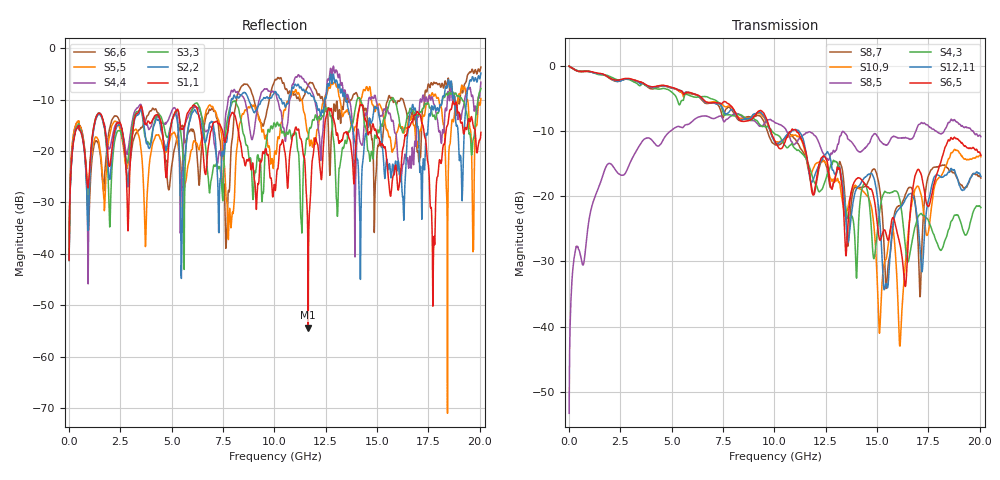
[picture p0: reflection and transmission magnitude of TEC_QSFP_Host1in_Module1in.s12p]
!!  This file represents Tyco Electronics parts only.  Due to internal design and materials, it should not  !!
!!  be used for products manufactured by companies other than Tyco Electronics.  !!
!! FILE NAME: TEC_QSFP_Host1in_Module1in.s12p
!! PART DESCRIPTION: Tyco Electronics QSFP P/N 1761987-9
!! PCB DESCRIPTION: Host Board FR4 with 1.5 inch microstrip, Module Board FR4 with 1.5 inch microstrip
!! FILE DESCRIPTION: 12 Port, S-Parameter, Measured Channel
!! FILE REVISION: Revision 2, 3/12/2008
!! FILE FREQUENCY RANGE: DC to 20.05 GHz in 12.50 MHz frequency steps
!! PORT DEFINITIONS:
!! Port  1  ----->  Host	Pin 14, RX3+	Module  <-----  Port  2
!! Port  3  ----->  Host	Pin 15, RX3-	Module  <-----  Port  4
!! Port  5  ----->  Host	Pin 21, RX2-	Module  <-----  Port  6
!! Port  7  ----->  Host	Pin 22, RX2+	Module  <-----  Port  8
!! Port  9  ----->  Host	Pin 24, RX4-	Module  <-----  Port  10
!! Port  11  ----->  Host	Pin 25, RX4+	Module  <-----  Port  12
# HZ S MA R 50.00
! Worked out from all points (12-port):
!   1604 points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, 12.5 MHz to 20.05 GHz, reference 50 ohm
!   strongest paths, dB at 12.5 MHz, 5.025 GHz, 10.04 GHz, 15.05 GHz, 20.05 GHz:
!     S6,5: 0.0, -3.3, -11.7, -25.4, -13.7
!     S12,11: -0.1, -3.4, -11.8, -21.1, -17.0
!     S4,3: -0.1, -4.1, -10.5, -24.2, -21.8
!     S8,5: -53.3, -9.8, -8.7, -11.0, -10.9
!     S10,9: -0.1, -3.4, -11.6, -36.5, -13.9
!     S8,7: -0.1, -3.4, -12.1, -17.5, -17.2
!   lowest |S11| = -54.4 dB at 11.65 GHz (marker M1), VSWR 1.00, Z = 50.1 - j0.137 ohm
!   |S11| at or under -10 dB: start of sweep to end of sweep
